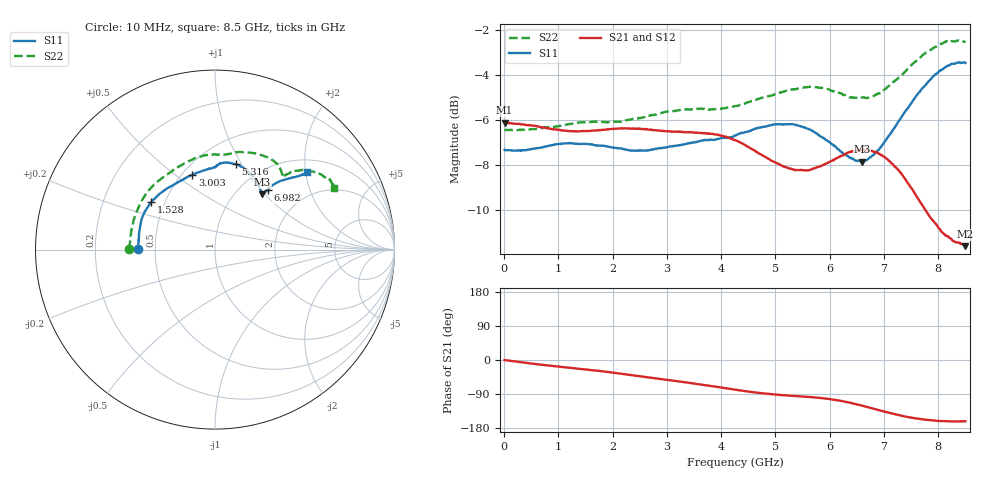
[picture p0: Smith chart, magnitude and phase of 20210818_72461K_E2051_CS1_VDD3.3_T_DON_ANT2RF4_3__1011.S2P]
!Agilent Technologies,E5071C,MY46417908,A.11.23
!Date: Wed Aug 18 14:34:29 2021
!Data & Calibration Information:
!Freq	S11:SOLT2(ON)	S21:SOLT2(ON)	S12:SOLT2(ON)	S22:SOLT2(ON)
!PortZ  Port1:50+j0  Port2:50+j0
!Above PortZ is port z conversion or system Z0 setting when saving the data.
!When reading, reference impedance value at option line is always used.
# Hz S dB R 50
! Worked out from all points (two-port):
!   1601 points, 10 MHz to 8.5 GHz, reference 50 ohm
!   highest |S21| = -6.13 dB at 10 MHz (marker M1); lowest = -11.6 dB at 8.5 GHz (marker M2)
!   |S21| within 3 dB of the highest: start of sweep to 7.533 GHz
!   lowest |S11| = -7.9 dB at 6.595 GHz (marker M3), VSWR 2.36, Z = 65.6 + j48.2 ohm
!   |S11| at or under -10 dB: nowhere
!   |S22| runs from -6.5 to -2.5 dB; largest |S21 - S12| = 0.0015
!   S11 on the Smith chart (normalised r, x): 10 MHz: 0.40, +0.00; 1.528 GHz: 0.42, +0.28; 3.003 GHz: 0.56, +0.58; 5.316 GHz: 0.75, +0.95; 6.982 GHz: 1.32, +1.09; 8.5 GHz: 1.30, +2.04
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1e7  -7.33 179.6  -6.13 -0.3  -6.12 -0.3  -6.43 179.6
7.847125e8  -7.18 161.8  -6.37 -14.1  -6.36 -14.1  -6.34 159.1
1.426769e9  -7.07 146.0  -6.50 -23.7  -6.50 -23.7  -6.11 140.3
1.527588e9  -7.07 143.4  -6.50 -25.3  -6.50 -25.3  -6.10 137.4
2.180256e9  -7.29 127.3  -6.38 -36.7  -6.38 -36.7  -6.07 119.8
2.843538e9  -7.27 110.6  -6.47 -49.5  -6.47 -49.5  -5.74 104.5
3.002725e9  -7.22 106.9  -6.51 -52.5  -6.50 -52.5  -5.63 101.4
3.597025e9  -6.95 95.5  -6.59 -64.0  -6.58 -64.0  -5.51 90.6
4.255e9  -6.71 89.4  -6.91 -78.2  -6.90 -78.2  -5.39 82.2
4.785625e9  -6.31 85.5  -7.62 -88.2  -7.62 -88.2  -5.00 75.3
5.31625e9  -6.19 76.2  -8.20 -94.6  -8.21 -94.5  -4.65 64.8
5.671769e9  -6.48 67.6  -8.20 -98.1  -8.21 -98.1  -4.54 57.9
6.101575e9  -7.18 56.6  -7.74 -105.3  -7.76 -105.4  -4.75 51.3
6.425256e9  -7.74 50.9  -7.41 -114.6  -7.41 -114.7  -5.01 47.5
6.595056e9  -7.86 49.4  -7.34 -120.4  -7.34 -120.5  -5.01 47.3
6.982412e9  -7.08 48.6  -7.62 -135.2  -7.63 -135.2  -4.71 46.2
7.088538e9  -6.71 48.6  -7.81 -139.2  -7.83 -139.2  -4.49 45.7
7.359156e9  -5.74 46.9  -8.53 -148.2  -8.53 -148.3  -3.94 43.7
7.550181e9  -5.09 44.6  -9.20 -153.4  -9.19 -153.4  -3.46 41.4
7.77835e9  -4.41 42.2  -10.07 -157.8  -10.05 -157.9  -2.99 37.5
8.11795e9  -3.68 40.1  -11.10 -161.4  -11.08 -161.4  -2.54 31.7
8.5e9  -3.47 40.0  -11.62 -161.7  -11.60 -161.8  -2.56 27.4
